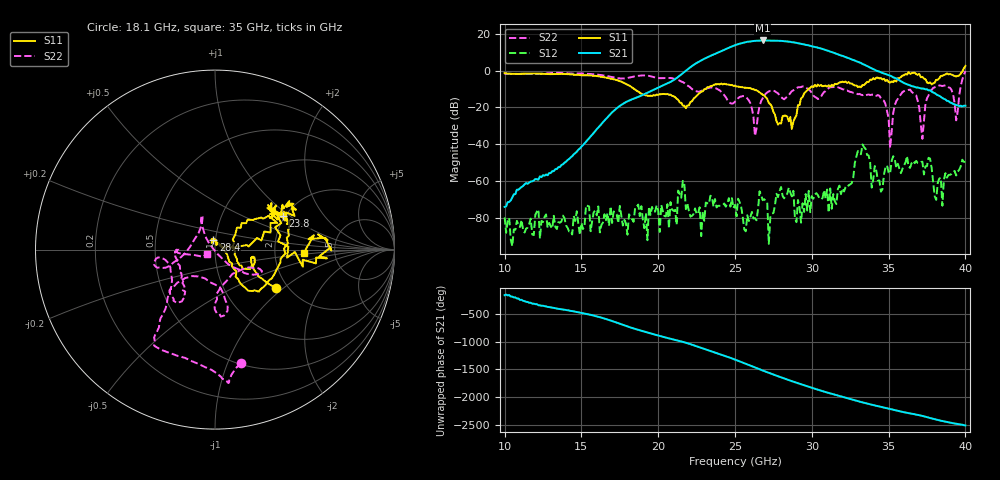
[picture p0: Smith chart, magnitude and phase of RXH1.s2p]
!Keysight Technologies,M9808A,MY58100618,A.14.70.03
!Date: Monday, February 27, 2023 13:42:53
!Correction: S11(Cdelta 2-Port  )
!S21(Cdelta 2-Port  )
!S12(Cdelta 2-Port  )
!S22(Cdelta 2-Port  )
!S2P File: Measurements: S11, S21, S12, S22:
# Hz S  RI  R 50
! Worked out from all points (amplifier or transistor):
!   301 points, 10 GHz to 40 GHz, reference 50 ohm
!   highest |S21| = 16.4 dB at 26.8 GHz (marker M1)
!   |S21| within 3 dB of that: 24.87 GHz to 29.93 GHz (5.058 GHz wide, 18.5 % of centre)
!   unconditionally stable (mu >= 1): start of sweep to 39.82 GHz
!   at 15 GHz: K = 99475.34, MAG = -32.3 dB, |S12| = -82.7 dB
!   at 25 GHz: K = 373.61, MAG = 14.7 dB, |S12| = -72.9 dB
!   at 40 GHz: K = -46.89, MSG = 15.3 dB, |S12| = -49.6 dB
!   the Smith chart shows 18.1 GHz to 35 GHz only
!   S11 on the Smith chart (normalised r, x): 18.1 GHz: 1.74, -0.88; 23.8 GHz: 1.95, +0.90; 28.4 GHz: 0.98, +0.11; 35 GHz: 2.94, -0.15
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1e10  -0.0203 0.8565  -0.000191 -5.11e-05  -9.88e-05 2.73e-05  0.7321 0.3613
1.5e10  0.7263 0.2066  -0.00458 -0.00723  -2.78e-05 -6.76e-05  0.6377 -0.5513
1.81e10  0.3383 -0.2131  0.1475 -0.0438  -5.21e-05 0.000114  0.1441 -0.6316
2e10  0.2142 -0.0467  -0.3417 -0.06  5.54e-05 0.000149  -0.1284 -0.6219
2.27e10  0.1811 0.1669  1.666 -0.7057  0.000183 6.21e-05  -0.2603 -0.075
2.38e10  0.3798 0.1894  -1.739 -2.427  0.000117 -0.000153  -0.3095 -0.1004
2.45e10  0.4076 0.11  -3.974 0.809  8.24e-05 0.000232  -0.1608 -0.013
2.5e10  0.3918 -0.0212  -2.26 4.368  -0.000188 0.000125  -0.0805 0.1209
2.55e10  0.3175 -0.1597  2.557 5.057  -9.35e-05 -5.68e-05  -0.0716 0.1905
2.6e10  0.2438 -0.2344  6.157 0.8642  -7.37e-05 7.42e-05  -0.0656 0.1122
2.63e10  0.1937 -0.2302  5.876 -2.706  -9.61e-05 -2.14e-05  -0.0139 0.00956
2.68e10  0.1345 -0.1772  1.223 -6.522  4.55e-06 -0.000301  0.1377 -0.1127
2.76e10  0.0622 -0.0186  -6.254 -2.005  0.000112 -0.000182  0.2516 -0.1095
2.84e10  -0.00924 0.0559  -2.928 5.527  0.000216 -0.000394  0.0493 -0.1905
2.88e10  0.0125 0.039  1.079 5.803  -0.000521 0.000153  0.00366 -0.2922
2.93e10  0.177 0.0255  4.493 2.991  -1.24e-05 7.27e-05  0.025 -0.3575
3e10  0.3464 0.149  3.99 -2.312  -6.71e-05 0.000382  0.0459 -0.2433
3.07e10  0.3095 0.214  -0.0448 -3.897  -0.000305 -0.00016  -0.1681 -0.1597
3.15e10  0.3841 0.2115  -2.75 -1.222  0.000235 -0.000156  -0.2315 -0.2846
3.27e10  0.3669 0.1937  -0.7283 1.815  -0.00101 -0.000713  -0.1774 -0.1767
3.5e10  0.4936 -0.0195  0.5378 -0.5316  -0.00135 0.00105  -0.0458 -0.0241
4e10  1.097 -0.7917  0.1091 0.0241  -0.00197 0.00266  0.4955 -0.8438
